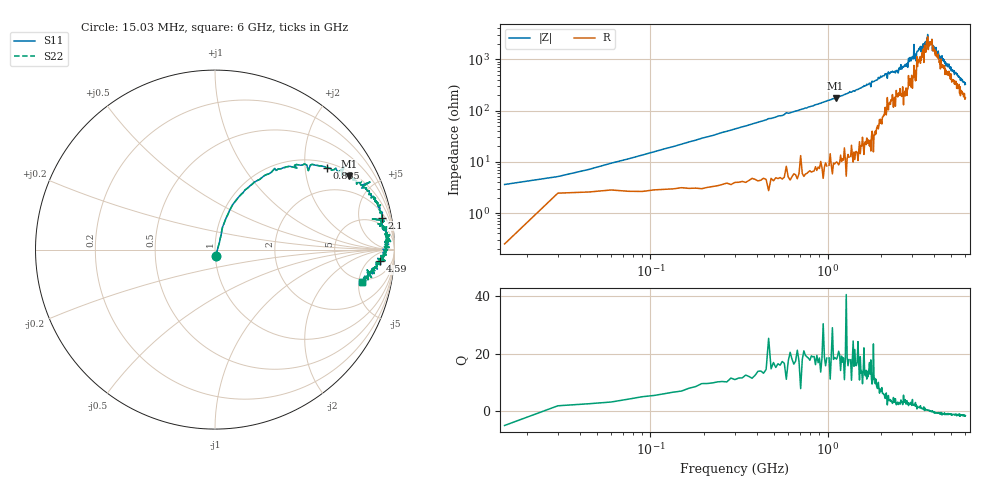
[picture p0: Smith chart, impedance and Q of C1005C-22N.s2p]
!	Network	Analyzer	HP8753E.07.74:	Oct	30	2002	Serial	No.	JP38451487
!	Hewlett-Packard
!	7	Sep	2009	8:57:29
!	Frequency	S11	S21	S12	S22
#	HZ	S	RI	R	50
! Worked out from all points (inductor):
!   400 points, 15.03 MHz to 6 GHz, reference 50 ohm
!   read as one part in series: L = 23.5 nH near 60.03 MHz
!   highest Q = 19.2 at 1.11 GHz (marker M1), where L = 25.3 nH
!   self-resonance near 3.786 GHz
!   S11 on the Smith chart (normalised r, x): 15.03 MHz: 1.00, -0.07; 855 MHz: 1.16, +2.60; 2.1 GHz: 3, +10; 4.59 GHz: 14, -12; 6 GHz: 4.52, -5.56
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1.502992e7  0.00356 -0.0358  0.996 0.0358  0.996 0.0358  0.00356 -0.0358
1.050295e8  0.0491 0.143  0.951 -0.143  0.951 -0.143  0.0491 0.143
2.550287e8  0.146 0.308  0.854 -0.308  0.854 -0.308  0.146 0.308
8.550257e8  0.622 0.455  0.378 -0.455  0.378 -0.455  0.622 0.455
1.020025e9  0.707 0.429  0.293 -0.429  0.293 -0.429  0.707 0.429
1.110024e9  0.746 0.409  0.254 -0.409  0.254 -0.409  0.746 0.409
2.01002e9  0.928 0.198  0.0718 -0.198  0.0718 -0.198  0.928 0.198
2.10002e9  0.929 0.178  0.071 -0.178  0.071 -0.178  0.929 0.178
3.015015e9  0.973 0.0814  0.0275 -0.0814  0.0275 -0.0814  0.973 0.0814
3.060015e9  0.96 0.0734  0.0403 -0.0734  0.0403 -0.0734  0.96 0.0734
3.075015e9  0.978 0.0453  0.0217 -0.0453  0.0217 -0.0453  0.978 0.0453
3.105014e9  0.954 0.0791  0.0464 -0.0791  0.0464 -0.0791  0.954 0.0791
3.165014e9  0.948 0.0889  0.0523 -0.0889  0.0523 -0.0889  0.948 0.0889
3.345013e9  0.972 0.0468  0.0278 -0.0468  0.0278 -0.0468  0.972 0.0468
3.585012e9  0.948 0.0287  0.0523 -0.0287  0.0523 -0.0287  0.948 0.0287
3.675012e9  0.971 0.0126  0.0292 -0.0126  0.0292 -0.0126  0.971 0.0126
3.705011e9  0.944 0.0164  0.0557 -0.0164  0.0557 -0.0164  0.944 0.0164
3.885011e9  0.961 -9.16e-05  0.0393 9.16e-05  0.0393 9.16e-05  0.961 -9.16e-05
4.00501e9  0.953 -0.03  0.0465 0.03  0.0465 0.03  0.953 -0.03
4.590007e9  0.92 -0.0645  0.0801 0.0645  0.0801 0.0645  0.92 -0.0645
5.010005e9  0.895 -0.0967  0.105 0.0967  0.105 0.0967  0.895 -0.0967
6e9  0.82 -0.181  0.18 0.181  0.18 0.181  0.82 -0.181
